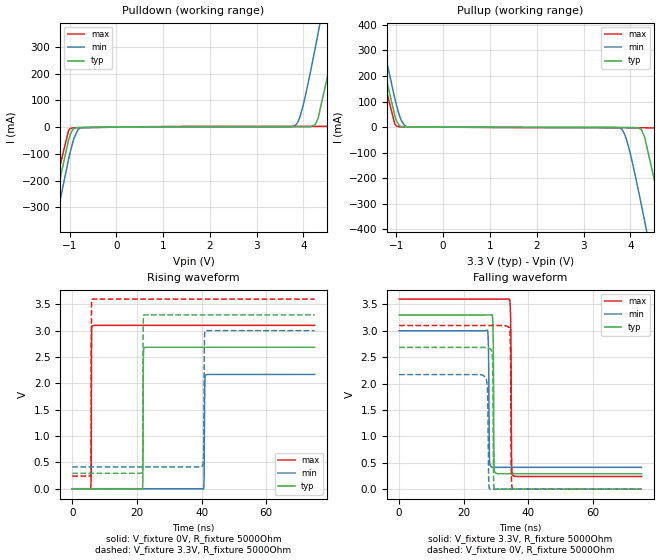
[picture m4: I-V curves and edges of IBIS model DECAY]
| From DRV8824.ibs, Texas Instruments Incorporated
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|   Model DECAY
[Model]   DECAY
Model_type   Output
Polarity   Non-Inverting
Vmeas = 1.65
Vref = 3.3
Cref = 15pF
Rref = 5000
|   typ   min   max
C_comp   0.1p   0.1p   0.1p
[Voltage Range]   3.3   3   3.6
[Temperature Range]   27   125   -40
[Pullup Reference]   3.3   3   3.6
[Pulldown Reference]   -0   -0   -0
[Power Clamp Reference]   3.3   3   3.6
[GND Clamp Reference]   -0   -0   -0
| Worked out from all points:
|   slope of the pulldown table from 0 to 0.495 V, typ, clamps not added: 530 ohm
|   slope of the pullup table from 0 to 0.495 V, typ, clamps not added: 1.12 kohm
|   falling waveform, V_fixture 3.3V, R_fixture 5000Ohm: 20-80 % time 163ps typ, 203ps min, 177ps max; typ from 3.3 V to 0.293 V
|   rising waveform, V_fixture 0V, R_fixture 5000Ohm: 20-80 % time 80.8ps typ, 138ps min, 64ps max; typ from 0 V to 2.69 V
|   rising waveform, V_fixture 3.3V, R_fixture 5000Ohm: 20-80 % time 86.3ps typ, 141ps min, 69.8ps max; typ from 0.293 V to 3.3 V
|   falling waveform, V_fixture 0V, R_fixture 5000Ohm: 20-80 % time 169ps typ, 262ps min, 172ps max; typ from 2.69 V to 0 V
[Pulldown]
|   Voltage   I(typ)   I(min)   I(max)
-3.3V     -2.228A    -2.299A    -2.187A
-1.855V   -808.9mA   -886.4mA   -762.9mA
-1.36V    -336.6mA   -417.3mA   -287.6mA
-983.4mV  -27.19mA   -92.96mA   -5.113mA
-686.4mV  -1.398mA   -1.184mA   -1.793mA
3.808V    1.96mA     4.807mA    2.694mA
4.244V    7.723mA    289.4mA    2.746mA
4.59V     255.9mA    610.3mA    4.79mA
4.719V    374.7mA    732.7mA    63.65mA
4.907V    552.7mA    913.2mA    225.6mA
5.224V    858.1mA    1.22A      525.3mA
6.59V     2.2A       2.561A     1.866A
[Pullup]
|   Voltage   I(typ)   I(min)   I(max)
-3.3V     2.21A      2.275A     2.173A
-1.855V   790.8mA    862.6mA    748.8mA
-1.34V    301.1mA    376.3mA    255.7mA
-993.3mV  22.63mA    82.24mA    3.703mA
-765.6mV  816.1uA    1.667mA    1.076mA
3.788V    -1.458mA   -4.878mA   -2.313mA
4.234V    -9.137mA   -302.6mA   -2.452mA
4.58V     -263.8mA   -624.2mA   -5.075mA
4.719V    -392.1mA   -756.2mA   -74.69mA
4.927V    -589.4mA   -956.1mA   -257.2mA
5.224V    -876.1mA   -1.244A    -539.2mA
6.59V     -2.218A    -2.585A    -1.88A
[Ramp]
R_load = 5000
|   typ   min   max
dV/dt_r   1.61123/8.07607e-11   1.30196/1.38303e-10   1.86063/6.39879e-11
dV/dt_f   1.80429/1.62843e-10   1.55196/2.03286e-10   2.01574/1.77103e-10
[Falling Waveform]
V_fixture = 3.3V
V_fixture_min = 3V
V_fixture_max = 3.6V
R_fixture = 5000Ohm
C_fixture = 0F
|   Time   V(typ)   V(min)   V(max)
0s        3.3V       3V         3.6V
27.36ns   3.301V     3.007V     3.6V
27.95ns   3.301V     589.1mV    3.6V
28.75ns   3.307V     417mV      3.6V
29.11ns   2.735V     414mV      3.6V
29.34ns   494mV      413.7mV    3.6V
29.9ns    305mV      413.7mV    3.6V
34.31ns   292.8mV    413.7mV    3.52V
35.14ns   292.8mV    413.6mV    262.2mV
75ns      292.8mV    413.4mV    240.4mV
[Rising Waveform]
V_fixture = 0V
V_fixture_min = 0V
V_fixture_max = 0V
R_fixture = 5000Ohm
C_fixture = 0F
|   Time   V(typ)   V(min)   V(max)
0s        1.383nV    3.282nV    -30.72nV
5.733ns   4.199uV    5.001uV    29.13mV
5.965ns   4.368uV    5.203uV    2.901V
6.211ns   4.548uV    5.417uV    3.092V
21.7ns    2.467mV    18.92uV    3.101V
21.99ns   2.505V     19.18uV    3.101V
22.28ns   2.677V     19.42uV    3.101V
40.59ns   2.685V     -8.095mV   3.101V
41.31ns   2.685V     2.16V      3.101V
75ns      2.685V     2.17V      3.101V
[Rising Waveform]
V_fixture = 3.3V
V_fixture_min = 3V
V_fixture_max = 3.6V
R_fixture = 5000Ohm
C_fixture = 0F
|   Time   V(typ)   V(min)   V(max)
0s        292.8mV    413.4mV    240.4mV
5.684ns   292.8mV    413.4mV    270.7mV
6.07ns    292.8mV    413.4mV    3.595V
21.57ns   314.6mV    413.4mV    3.6V
22.11ns   3.297V     413.4mV    3.6V
40.21ns   3.3V       427.6mV    3.6V
40.63ns   3.3V       668.5mV    3.6V
40.88ns   3.3V       2.793V     3.6V
41.13ns   3.3V       2.998V     3.6V
75ns      3.3V       3V         3.6V
[Falling Waveform]
|Gnd
V_fixture = 0V
V_fixture_min = 0V
V_fixture_max = 0V
R_fixture = 5000Ohm
C_fixture = 0F
|   Time   V(typ)   V(min)   V(max)
0s        2.685V     2.17V      3.101V
26.69ns   2.684V     2.117V     3.101V
28.45ns   2.639V     1.108mV    3.101V
28.93ns   2.363V     415.4uV    3.101V
29.37ns   25.27mV    -34.25uV   3.101V
34.06ns   -63.89uV   -30.72uV   3.057V
34.45ns   -63.27uV   -30.43uV   2.531V
34.68ns   -62.91uV   -30.26uV   319.5mV
35.14ns   -62.2uV    -29.91uV   3.311mV
75ns      1.513nV    3.277nV    1.324nV
